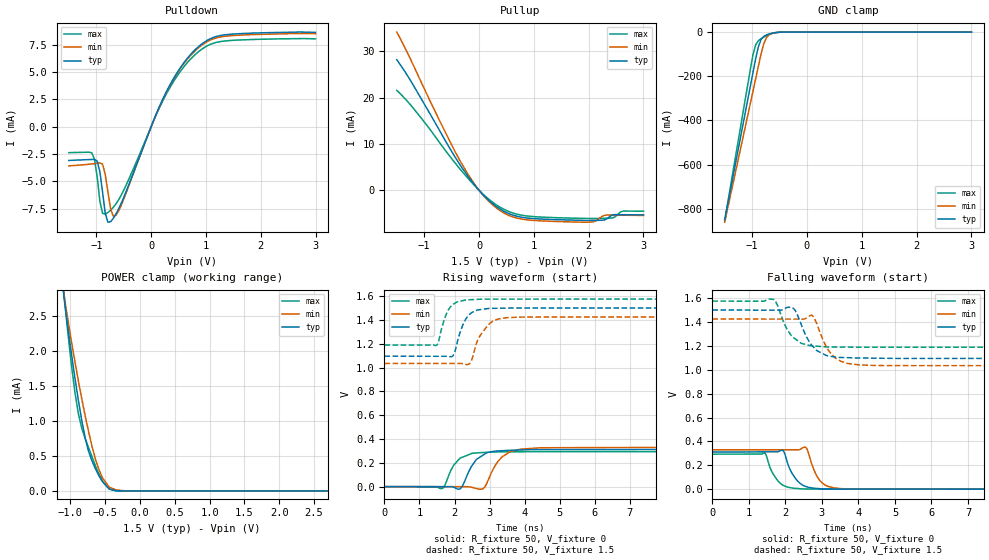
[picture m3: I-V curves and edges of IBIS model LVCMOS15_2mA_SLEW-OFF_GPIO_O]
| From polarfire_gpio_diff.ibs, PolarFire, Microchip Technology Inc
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|   Model LVCMOS15_2mA_SLEW-OFF_GPIO_O
[Model]   LVCMOS15_2mA_SLEW-OFF_GPIO_O
Model_type   Output
Polarity   Non-Inverting
Enable   Active-High
Vmeas =   0.75
Cref =   5p
Rref =   1M
|   typ   min   max
C_comp_pullup   2.605e-12   2.605e-12   2.76e-12
C_comp_pulldown  2.605e-12   2.605e-12   2.76e-12
[Temperature Range]  25C   100C   -40C
[Voltage Range]  1.5   1.425   1.575
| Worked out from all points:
|   slope of the pulldown table from 0 to 0.225 V, typ, clamps not added: 84.8 ohm
|   slope of the pullup table from 0 to 0.225 V, typ, clamps not added: 84.7 ohm
|   GND clamp passes 1 mA (typ) near -0.52 V on its own axis
|   POWER clamp passes 1 mA (typ) near -0.84 V on its own axis
|   rising waveform, R_fixture 50, V_fixture 0: 20-80 % time 421ps typ, 453ps min, 355ps max; typ from 0 V to 0.312 V
|   rising waveform, R_fixture 50, V_fixture 1.5: 20-80 % time 301ps typ, 392ps min, 273ps max; typ from 1.09 V to 1.5 V
|   falling waveform, R_fixture 50, V_fixture 0: 20-80 % time 324ps typ, 294ps min, 306ps max; typ from 0.312 V to 0 V
|   falling waveform, R_fixture 50, V_fixture 1.5: 20-80 % time 429ps typ, 417ps min, 402ps max; typ from 1.5 V to 1.09 V
[GND Clamp]
| Voltage   I(typ)   I(min)   I(max)
-1.5V     -849.7mA   -860.2mA   -853.5mA
-1.034V   -246.6mA   -324.3mA   -170.7mA
-984.4mV  -183.1mA   -267.7mA   -102.9mA
-935.2mV  -119.9mA   -211.2mA   -57.59mA
-885.9mV  -66.33mA   -154.7mA   -38.94mA
-836.7mV  -33.59mA   -99.09mA   -29.82mA
-787.5mV  -19.44mA   -53.53mA   -22.49mA
-738.3mV  -12.87mA   -24.95mA   -16.13mA
-689.1mV  -8.545mA   -11.57mA   -10.81mA
-590.6mV  -2.947mA   -3.067mA   -3.621mA
-393.7mV  -37.64uA   -63.17uA   -40.12uA
3V        0A         0A         0A
[POWER Clamp]
| Voltage   I(typ)   I(min)   I(max)
-1.5V     10.9mA     9.757mA    12.4mA
-1.181V   3.55mA     3.502mA    3.75mA
-1.083V   2.694mA    2.748mA    2.703mA
-984.4mV  1.956mA    2.133mA    1.792mA
-935.2mV  1.615mA    1.848mA    1.408mA
-836.7mV  1.007mA    1.316mA    894.8uA
-738.3mV  562.1uA    843.7uA    616.9uA
-639.8mV  314.2uA    451.1uA    357.6uA
-541.4mV  134.7uA    190.1uA    142.2uA
-443mV    26.83uA    53.65uA    28.29uA
-196.9mV  138.9nA    426.2nA    8.47nA
3V        0A         0A         0A
[Pullup]
| Voltage   I(typ)   I(min)   I(max)
-1.5V     28.19mA    34.17mA    21.6mA
-1.181V   22.35mA    26.59mA    17.48mA
-344.5mV  5.472mA    6.34mA     4.563mA
0V        -138.7nA   4.951uA    13.18uA
328.1mV   -3.607mA   -3.914mA   -3.24mA
656.2mV   -5.497mA   -5.895mA   -5.049mA
1.172V    -6.228mA   -6.627mA   -5.808mA
2.041V    -6.508mA   -6.859mA   -6.092mA
2.288V    -6.404mA   -5.405mA   -6.043mA
2.386V    -5.668mA   -5.349mA   -6.014mA
2.632V    -5.269mA   -5.385mA   -4.483mA
3V        -5.318mA   -5.433mA   -4.52mA
[Pulldown]
| Voltage   I(typ)   I(min)   I(max)
-1.5V     -3.075mA   -3.568mA   -2.36mA
-1.083V   -2.985mA   -3.394mA   -2.374mA
-984.4mV  -3.121mA   -3.333mA   -4.527mA
-885.9mV  -5.948mA   -3.405mA   -7.916mA
-836.7mV  -7.901mA   -4.365mA   -7.982mA
-738.3mV  -8.674mA   -7.499mA   -7.624mA
-689.1mV  -8.363mA   -8.187mA   -7.362mA
-590.6mV  -7.483mA   -7.679mA   -6.66mA
281.2mV   3.23mA     3.185mA    3.035mA
843.8mV   7.243mA    7.142mA    6.783mA
1.359V    8.423mA    8.286mA    7.857mA
3V        8.641mA    8.518mA    8.044mA
[Ramp]
dV/dt_r   0.187103/0.420555n  0.197479/0.453461n  0.175927/0.355148n
dV/dt_f   0.242793/0.428966n  0.234428/0.417463n  0.231628/0.401737n
R_load = 50
[Rising Waveform]
R_fixture = 50
V_fixture = 0
V_fixture_min = 0
V_fixture_max = 0
| Time   V(typ)   V(min)   V(max)
0s        23.55nV    32.77nV    32.21nV
1.662ns   -855uV     15.96uV    -14.22mV
1.982ns   -5.876mV   19.03uV    182.5mV
2.153ns   -19.46mV   20.67uV    237.4mV
2.51ns    181mV      -6.772mV   280.4mV
2.829ns   267.6mV    -14.81mV   286.6mV
3.154ns   297.9mV    173.7mV    290.7mV
3.347ns   301.4mV    247.4mV    292.1mV
3.873ns   307.8mV    314.3mV    292.8mV
10ns      311.8mV    329.1mV    293.2mV
[Rising Waveform]
R_fixture = 50
V_fixture = 1.5
V_fixture_min = 1.425
V_fixture_max = 1.575
| Time   V(typ)   V(min)   V(max)
0s        1.095V     1.034V     1.189V
1.484ns   1.095V     1.034V     1.186V
1.745ns   1.095V     1.034V     1.433V
1.936ns   1.093V     1.034V     1.525V
2.331ns   1.411V     1.025V     1.568V
2.473ns   1.457V     1.051V     1.57V
2.658ns   1.483V     1.228V     1.572V
2.82ns    1.49V      1.306V     1.574V
3.347ns   1.498V     1.413V     1.575V
10ns      1.5V       1.425V     1.575V
[Falling Waveform]
R_fixture = 50
V_fixture = 0
V_fixture_min = 0
V_fixture_max = 0
| Time   V(typ)   V(min)   V(max)
0s        311.8mV    329.1mV    293.2mV
1.43ns    312.3mV    329.4mV    302.6mV
1.659ns   312.3mV    329.4mV    130.5mV
1.936ns   322.5mV    329.5mV    32.8mV
2.223ns   113.2mV    329.5mV    7.608mV
2.567ns   21.1mV     346.6mV    1.613mV
2.795ns   7.613mV    152.9mV    819uV
2.91ns    4.704mV    85.84mV    418.6uV
3.324ns   745.7uV    11.16mV    -29.25uV
10ns      1.291uV    4.205uV    103.4nV
[Falling Waveform]
R_fixture = 50
V_fixture = 1.5
V_fixture_min = 1.425
V_fixture_max = 1.575
| Time   V(typ)   V(min)   V(max)
0s        1.5V       1.425V     1.575V
1.691ns   1.499V     1.424V     1.587V
2.049ns   1.522V     1.424V     1.337V
2.228ns   1.512V     1.424V     1.268V
2.664ns   1.231V     1.45V      1.203V
2.78ns    1.187V     1.438V     1.2V
3.193ns   1.115V     1.156V     1.191V
3.367ns   1.106V     1.098V     1.19V
3.716ns   1.101V     1.052V     1.19V
10ns      1.095V     1.034V     1.189V
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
